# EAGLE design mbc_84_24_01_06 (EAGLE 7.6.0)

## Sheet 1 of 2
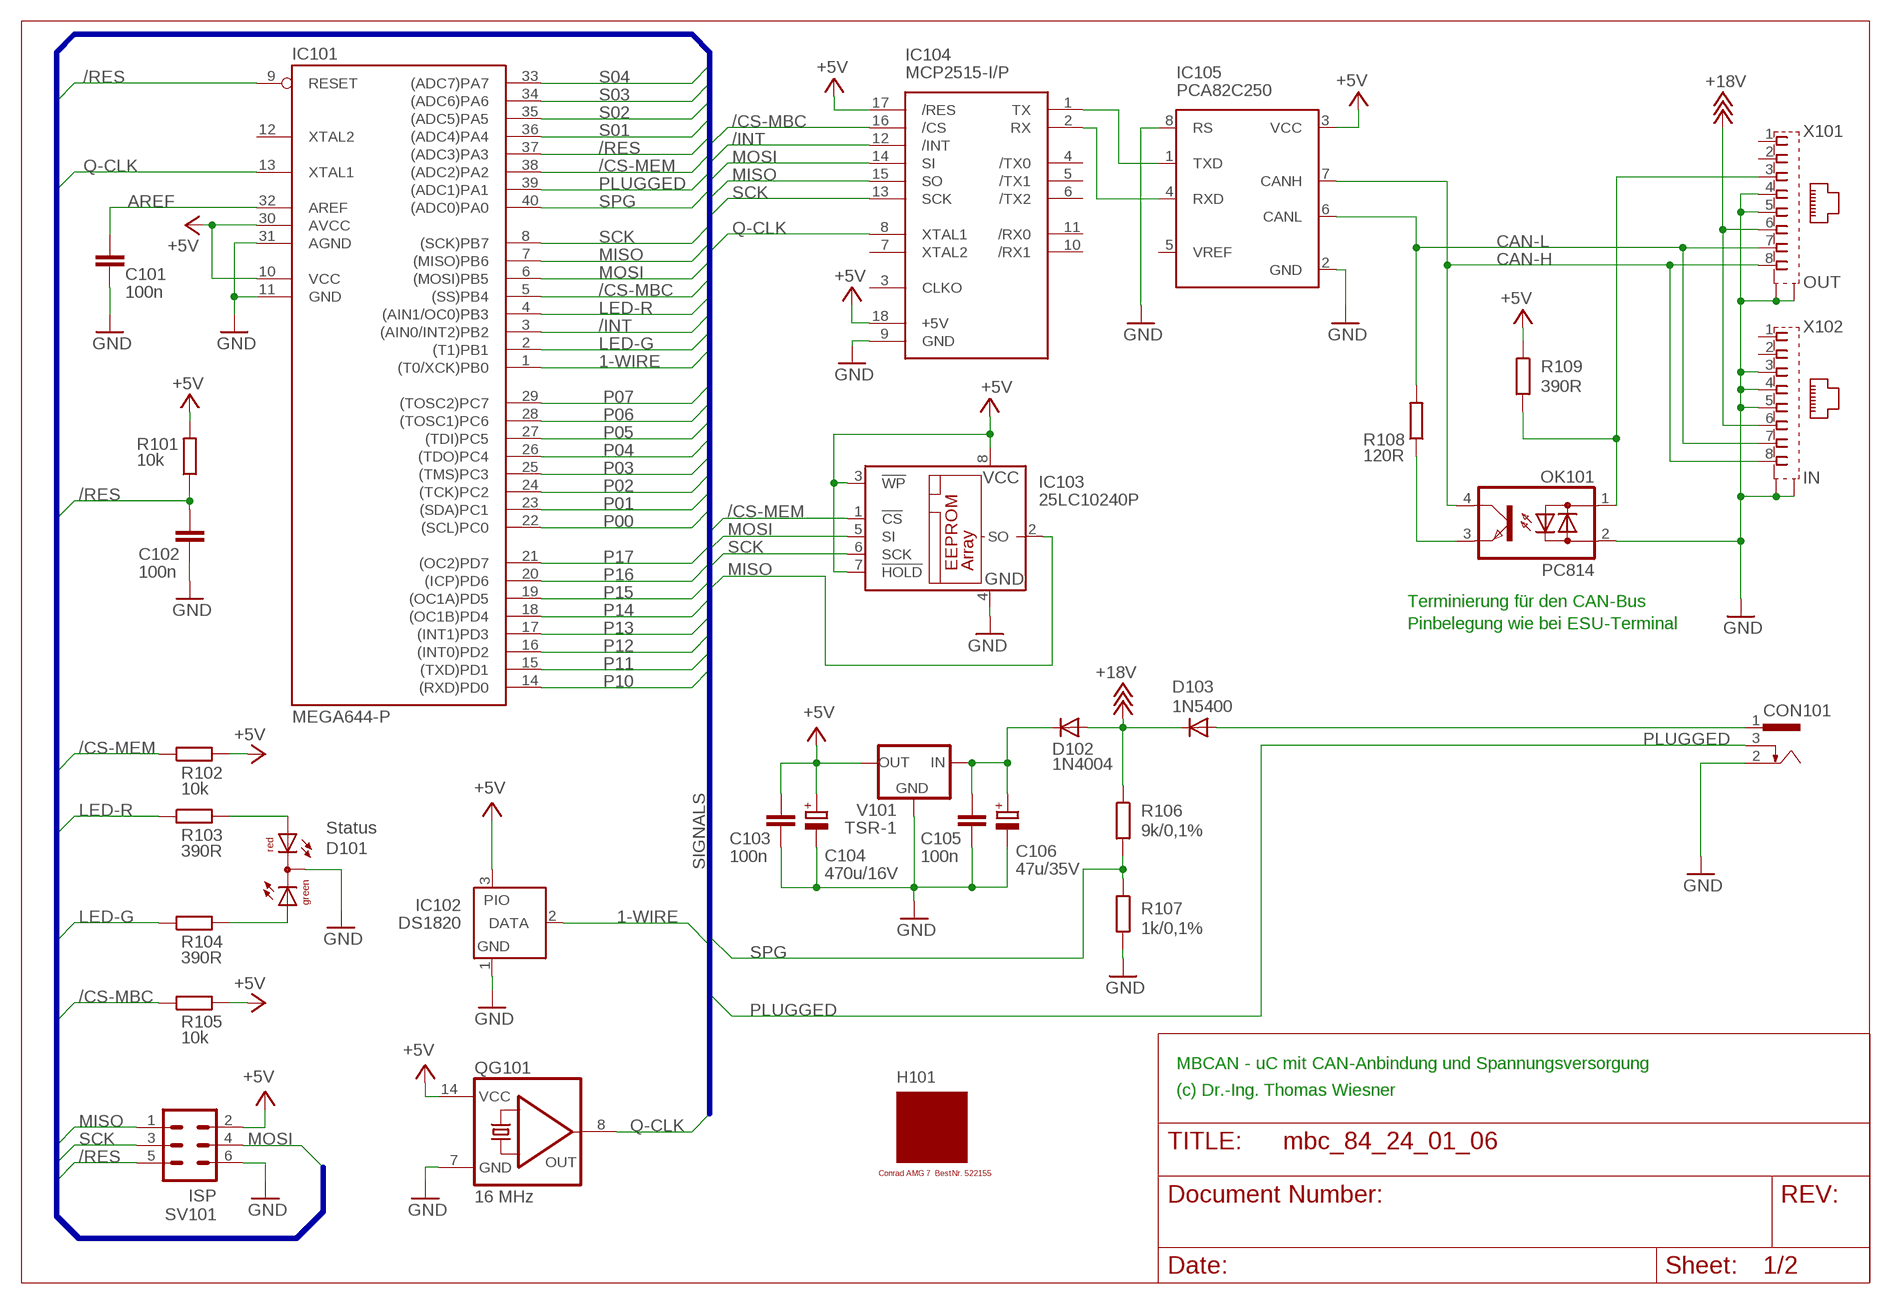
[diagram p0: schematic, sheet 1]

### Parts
C101  100n  C-EU025-025X050  [C025-025X050]
C102  100n  C-EU025-025X050  [C025-025X050]
C103  100n  C-EU025-025X050  [C025-025X050]
C104  470u/16V  CPOL-EUE3.5-8  [E3,5-8]
C105  100n  C-EU025-025X050  [C025-025X050]
C106  47u/35V  CPOL-EUE2.5-7  [E2,5-7]
CON101  POWER-JACK  [POWER-JACK]
D101  Status  DUOLED5MM  [DUOLED5MM]
D102  1N4004  [DO41-10]
D103  1N5400  [DO201-15]
H101  MODULGEHÄUSE-AMG-7  [MODULGEHÄUSE-1]
IC101  MEGA644-P  MEGA323-P  [DIL40]
IC102  DS1820  DS2405  [TO92-]
IC103  25LC10240P  25LC040P  [DIL8]
IC104  MCP2515-I/P  MCP2510-I/P  [DIL18]
IC105  PCA82C250  [DIL08]
OK101  PC814  [DIL04]
QG101  16 MHz  QG5860  [DIL14S]
R101  10k  R-EU_0207/10  [0207/10]
R102  10k  R-EU_0207/10  [0207/10]
R103  390R  R-EU_0207/10  [0207/10]
R104  390R  R-EU_0207/10  [0207/10]
R105  10k  R-EU_0207/10  [0207/10]
R106  9k/0,1%  R-EU_0207/10  [0207/10]
R107  1k/0,1%  R-EU_0207/10  [0207/10]
R108  120R  R-EU_0207/10  [0207/10]
R109  390R  R-EU_0207/10  [0207/10]
SV101  ISP  ML6  [ML6]
V101  TSR-1  [TRACO-TSR-1]
X101  OUT  0446200002  [0446200002]
X102  IN  0446200002  [0446200002]

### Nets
1-WIRE: IC101.1((T0/XCK)PB0) IC102.2(DATA)
+5V: C103.1 C104.+ IC101.10(VCC) IC101.30(AVCC) IC102.3(PIO) IC103.3(!WP) IC103.7(!HOLD) IC103.8(VCC) IC104.17(/RES) IC104.18(+5V) IC105.3(VCC) QG101.14(VCC) R101.2 R102.2 R105.2 R109.1 SV101.2 V101.OUT ; also sheet 2
+18V: D102.A D103.C R106.1 X101.6 X102.6 ; also sheet 2
/CS-MBC: IC101.5((SS)PB4) IC104.16(/CS) R105.1
/CS-MEM: IC101.38((ADC2)PA2) IC103.1(!CS) R102.1
/INT: IC101.3((AIN0/INT2)PB2) IC104.12(/INT)
/RES: C102.1 IC101.9(RESET) IC101.37((ADC3)PA3) R101.1 SV101.5
AREF: C101.1 IC101.32(AREF)
CAN-H: IC105.7(CANH) OK101.4(C) X101.8 X102.8
CAN-L: IC105.6(CANL) R108.2 X101.7 X102.7
GND: C101.2 C102.2 C103.2 C104.- C105.2 C106.- CON101.2 D101.K(C) IC101.11(GND) IC101.31(AGND) IC102.1(GND) IC103.4(GND) IC104.9(GND) IC105.2(GND) IC105.8(RS) OK101.2(AC2) QG101.7(GND) R107.2 SV101.6 V101.GND X101.4 X101.5 X101.S@1(S1) X101.S@2(S2) X102.3 X102.4 X102.5 X102.S@1(S1) X102.S@2(S2) ; also sheet 2
LED-G: IC101.2((T1)PB1) R104.1
LED-R: IC101.4((AIN1/OC0)PB3) R103.1
MISO: IC101.7((MISO)PB6) IC103.2(SO) IC104.15(SO) SV101.1
MOSI: IC101.6((MOSI)PB5) IC103.5(SI) IC104.14(SI) SV101.4
N$1: IC104.1(TX) IC105.1(TXD)
N$2: IC104.2(RX) IC105.4(RXD)
N$3: OK101.3(E) R108.1
N$5: OK101.1(AC1) R109.2 X101.3
N$6: C105.1 C106.+ D102.C V101.IN
N$9: D101.AR R103.2
N$13: D101.AG R104.2
P00: IC101.22((SCL)PC0) ; also sheet 2
P01: IC101.23((SDA)PC1) ; also sheet 2
P02: IC101.24((TCK)PC2) ; also sheet 2
P03: IC101.25((TMS)PC3) ; also sheet 2
P04: IC101.26((TDO)PC4) ; also sheet 2
P05: IC101.27((TDI)PC5) ; also sheet 2
P06: IC101.28((TOSC1)PC6) ; also sheet 2
P07: IC101.29((TOSC2)PC7) ; also sheet 2
P10: IC101.14((RXD)PD0) ; also sheet 2
P11: IC101.15((TXD)PD1) ; also sheet 2
P12: IC101.16((INT0)PD2) ; also sheet 2
P13: IC101.17((INT1)PD3) ; also sheet 2
P14: IC101.18((OC1B)PD4) ; also sheet 2
P15: IC101.19((OC1A)PD5) ; also sheet 2
P16: IC101.20((ICP)PD6) ; also sheet 2
P17: IC101.21((OC2)PD7) ; also sheet 2
PLUGGED: CON101.3 IC101.39((ADC1)PA1)
Q-CLK: IC101.13(XTAL1) IC104.8(XTAL1) QG101.8(OUT)
S01: IC101.36((ADC4)PA4) ; also sheet 2
S02: IC101.35((ADC5)PA5) ; also sheet 2
S03: IC101.34((ADC6)PA6) ; also sheet 2
S04: IC101.33((ADC7)PA7) ; also sheet 2
SCK: IC101.8((SCK)PB7) IC103.6(SCK) IC104.13(SCK) SV101.3
SPG: IC101.40((ADC0)PA0) R106.2 R107.1
V-NETZTEIL1: CON101.1 D103.A
Unconnected: IC101.12(XTAL2) IC104.3(CLKO) IC104.4(/TX0) IC104.5(/TX1) IC104.6(/TX2) IC104.7(XTAL2) IC104.10(/RX1) IC104.11(/RX0) IC105.5(VREF) X101.1 X101.2 X102.1 X102.2

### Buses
SIGNALS

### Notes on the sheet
- Terminierung für den CAN-Bus
- Pinbelegung wie bei ESU-Terminal
- MBCAN - uC mit CAN-Anbindung und Spannungsversorgung
- (c) Dr.-Ing. Thomas Wiesner

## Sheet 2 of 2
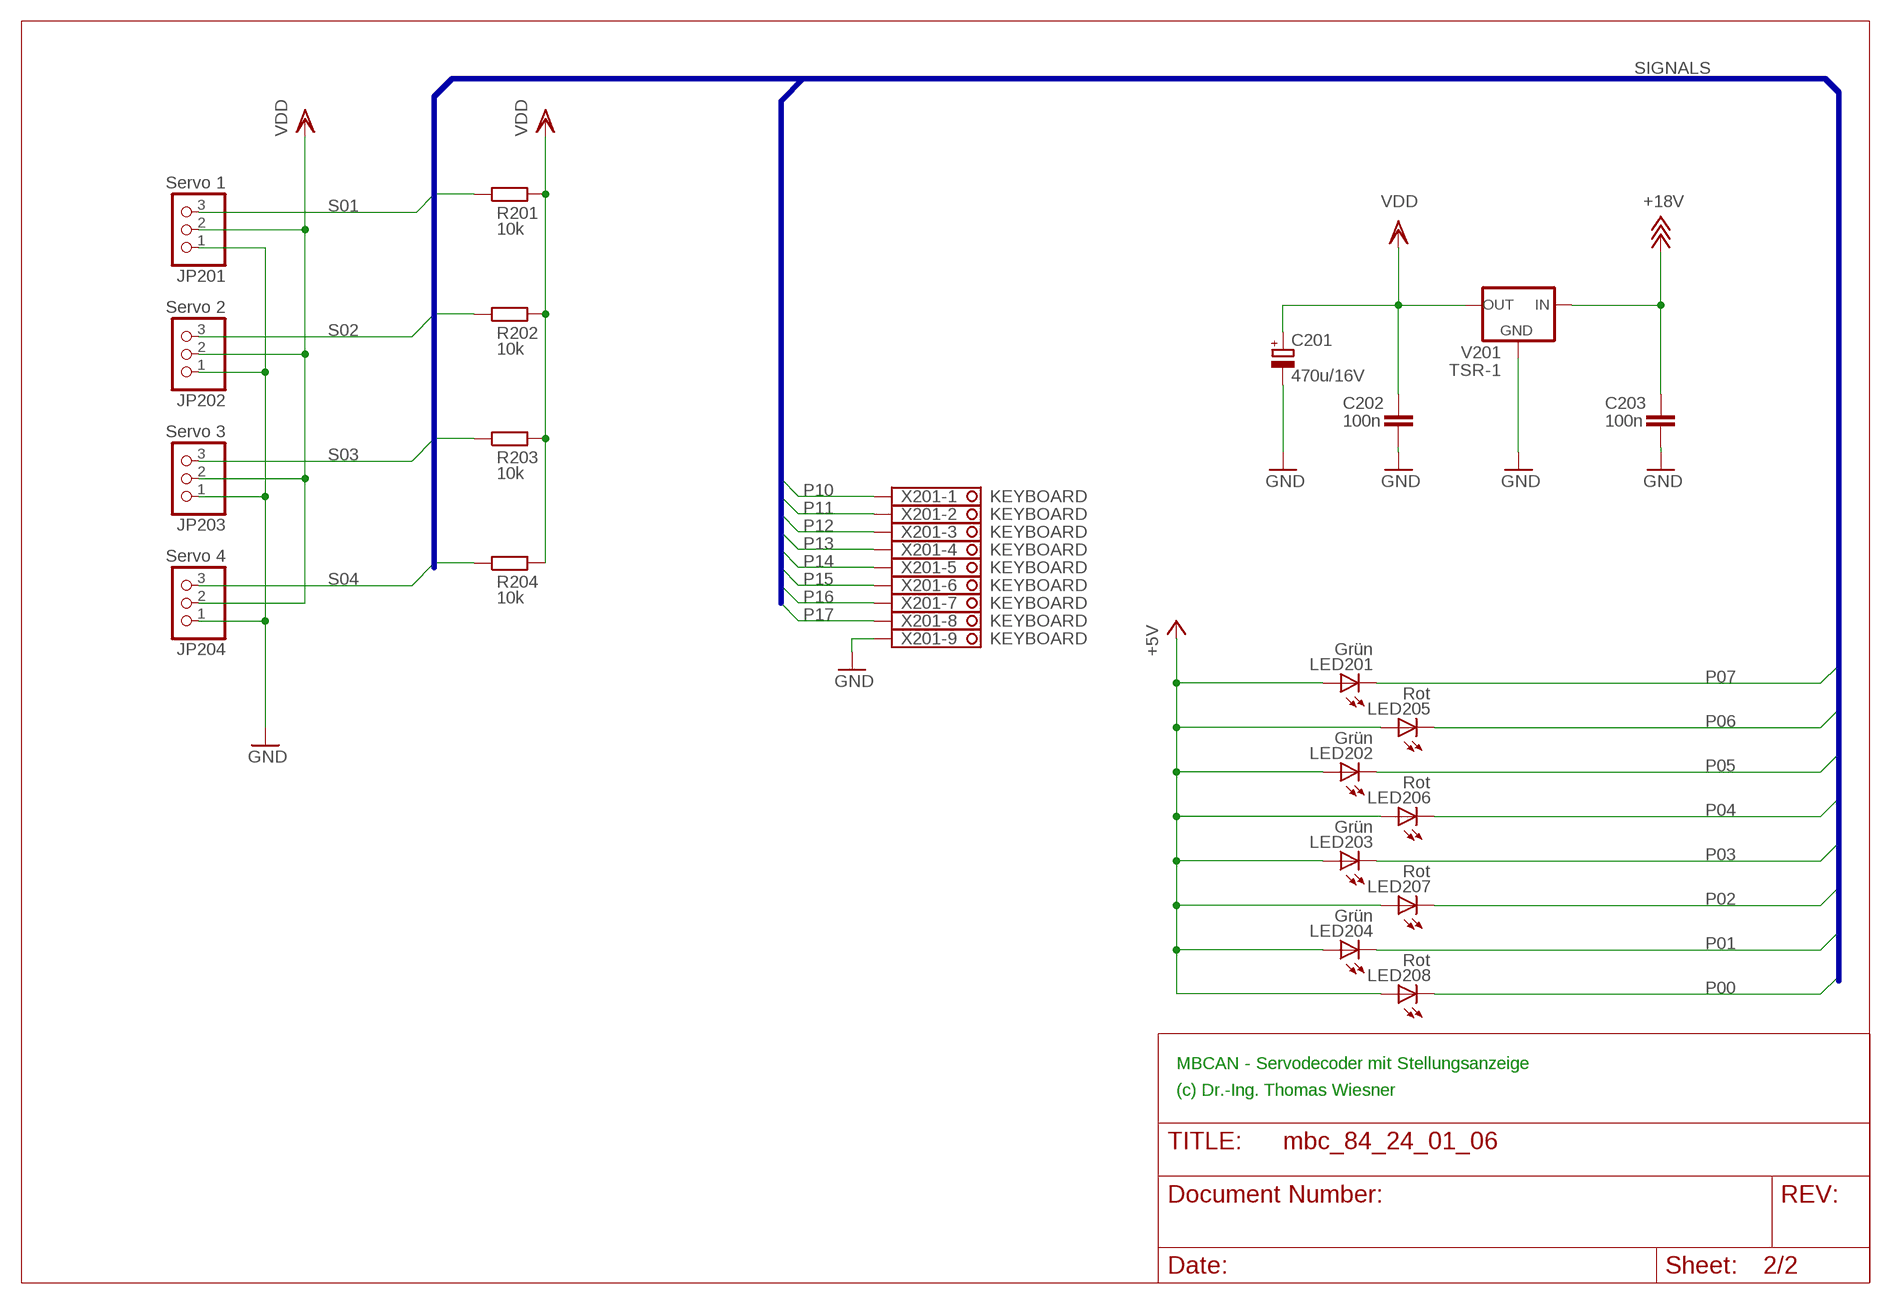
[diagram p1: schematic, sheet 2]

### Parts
C201  470u/16V  CPOL-EUE3.5-8  [E3,5-8]
C202  100n  C-EU025-025X050  [C025-025X050]
C203  100n  C-EU025-025X050  [C025-025X050]
JP201  Servo 1  PINHD-1X3  [1X03]
JP202  Servo 2  PINHD-1X3  [1X03]
JP203  Servo 3  PINHD-1X3  [1X03]
JP204  Servo 4  PINHD-1X3  [1X03]
LED201  Grün  LED3MM  [LED3MM]
LED202  Grün  LED3MM  [LED3MM]
LED203  Grün  LED3MM  [LED3MM]
LED204  Grün  LED3MM  [LED3MM]
LED205  Rot  LED3MM  [LED3MM]
LED206  Rot  LED3MM  [LED3MM]
LED207  Rot  LED3MM  [LED3MM]
LED208  Rot  LED3MM  [LED3MM]
R201  10k  R-EU_0207/10  [0207/10]
R202  10k  R-EU_0207/10  [0207/10]
R203  10k  R-EU_0207/10  [0207/10]
R204  10k  R-EU_0207/10  [0207/10]
V201  TSR-1  [TRACO-TSR-1]
X201  KEYBOARD  1751316  [1751316]

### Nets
+5V: LED201.A LED202.A LED203.A LED204.A LED205.A LED206.A LED207.A LED208.A ; also sheet 1
+18V: C203.1 V201.IN ; also sheet 1
GND: C201.- C202.2 C203.2 JP201.1 JP202.1 JP203.1 JP204.1 V201.GND X201.9 ; also sheet 1
P00: LED208.K(C) ; also sheet 1
P01: LED204.K(C) ; also sheet 1
P02: LED207.K(C) ; also sheet 1
P03: LED203.K(C) ; also sheet 1
P04: LED206.K(C) ; also sheet 1
P05: LED202.K(C) ; also sheet 1
P06: LED205.K(C) ; also sheet 1
P07: LED201.K(C) ; also sheet 1
P10: X201.1 ; also sheet 1
P11: X201.2 ; also sheet 1
P12: X201.3 ; also sheet 1
P13: X201.4 ; also sheet 1
P14: X201.5 ; also sheet 1
P15: X201.6 ; also sheet 1
P16: X201.7 ; also sheet 1
P17: X201.8 ; also sheet 1
S01: JP201.3 R201.1 ; also sheet 1
S02: JP202.3 R202.1 ; also sheet 1
S03: JP203.3 R203.1 ; also sheet 1
S04: JP204.3 R204.1 ; also sheet 1
VDD: C201.+ C202.1 JP201.2 JP202.2 JP203.2 JP204.2 R201.2 R202.2 R203.2 R204.2 V201.OUT

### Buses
SIGNALS

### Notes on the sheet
- MBCAN - Servodecoder mit Stellungsanzeige
- (c) Dr.-Ing. Thomas Wiesner

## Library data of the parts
C101-C103 C105 C202 C203 = rcl:C-EU: CAPACITOR, European symbol
C104 C106 C201 = rcl:CPOL-EU: POLARIZED CAPACITOR, European symbol
CON101 = mbc:POWER-JACK
D101 = led:DUOLED5MM: DUO LED 2 colors, 5 mm, round
D102 = diode:1N4004: DIODE
D103 = diode:1N5400: DIODE
H101 = mbc:MODULGEHÄUSE-AMG-7: Gehäuse
IC101 = atmel:MEGA323-P: MICROCONTROLLER 32 Kbytes FLASH 2 Kbytes SRAM 1 Kbytes EEPROM USART 8-channel 10 bit ADC Source: avr.lbr; OC_FARNELL: unknown; OC_NEWARK: unknown
IC102 = maxim:DS2405: Addressable Switch DALLAS Semiconductor; MF: DALLAS SEMICONDUCTOR; MPN: DS2405; OC_FARNELL: 1188025; OC_NEWARK: 06F4645
IC103 = microchip:25*: Serial EEPROM 4K/ 8K , SPI bus; MF: MICROCHIP; MPN: 25LC040/P; OC_FARNELL: 9758100; OC_NEWARK: 96K4091
IC104 = mbc:MCP2510: BASIC-CAN 2.0a Controller Stand-alone CAN controller von Microchip
IC105 = micro-philips:PCA82C250: CAN CONTROLLER INTERFACE; OC_FARNELL: 3692358; OC_NEWARK: unknown
JP201-JP204 = pinhead:PINHD-1X3: PIN HEADER
LED201-LED208 = led:LED: LED
OK101 = optocoupler:PC814: SHARP OPTO COUPLER; OC_FARNELL: 9707662; OC_NEWARK: unknown
QG101 = crystal:QG5860: CRYSTAL RESONATOR; OC_FARNELL: unknown; OC_NEWARK: unknown
R101-R109 R201-R204 = resistor:R-EU_: RESISTOR, European symbol
SV101 = con-ml:ML6: HARTING; OC_FARNELL: unknown; OC_NEWARK: unknown
V101 V201 = mbc:TSR-1: Spannungsregler Hersteller: TRACO Typ: TSR-1 5V: TSR 1-2450 Spg: 5V Strom: 1A Reichelt TSR 1-2450
X101 X102 = mbc:0446200002: RJ-45 INVERTED MODULAR JACK ASSEMBLY WITH RJ-11 KEEPOUT FEATURE Source: Data sheet MOLEX 0446200002 BUCHSE, RJ45, GESCHIRMT Source: Farnell; MF: MOLEX; MPN: 0446200002; OC_FARNELL: 9251910
X201 = con-phoenix-350:1751316: MKDS 1/ 9-3,5 Printklemme Nennstrom: 10 A Bemessungsspannung: 160 V Raster: 3,5 mm Polzahl: 9 Montageart: Löten Anschlussart: Schraubanschluss Anschlussrichtung vom Leiter zur Platine: 0° Source: http://eshop.phoenixcontact.com .. 1751316.pdf; OC_FARNELL: unknown; OC_NEWARK: unknown

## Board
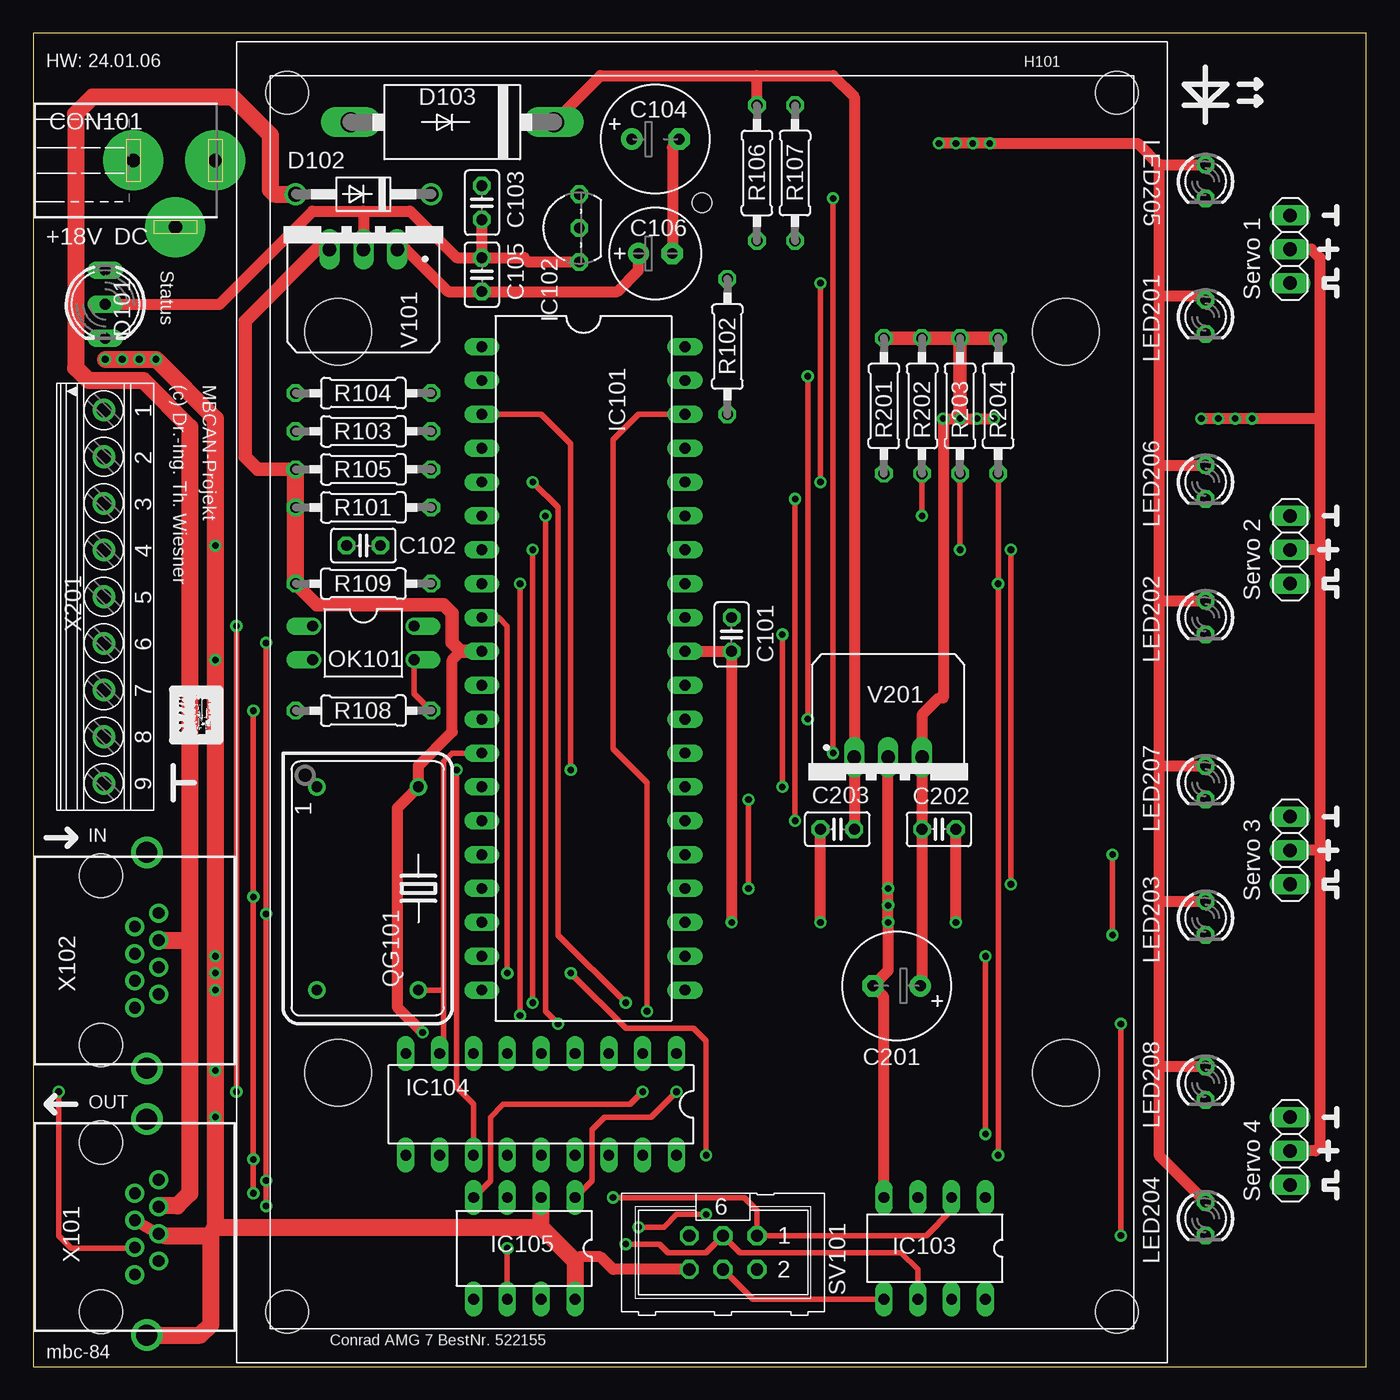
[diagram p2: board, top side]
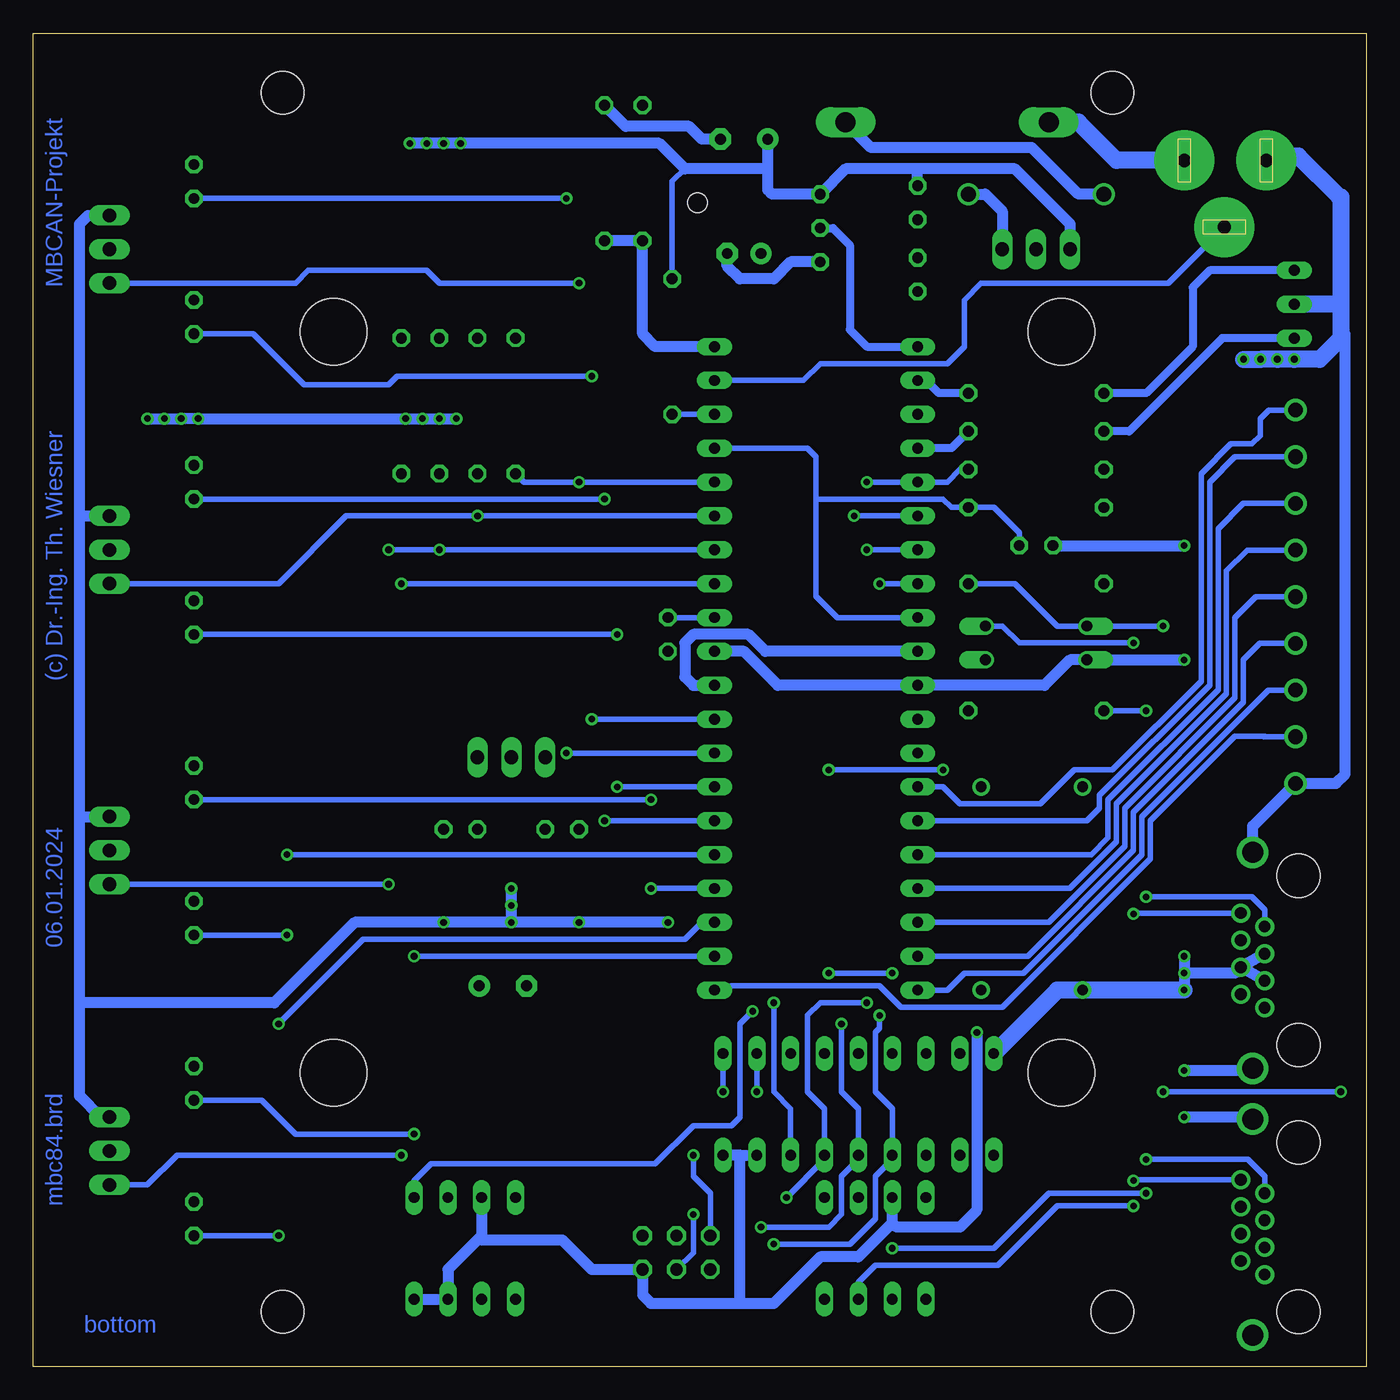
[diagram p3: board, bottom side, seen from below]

Size 100 x 99.99 mm. Coordinates in mm from the lower left corner, seen from the top.
Outline: 0,99.99 0,0 100,0 100,99.99 0,99.99
Copper layers (1*16): Top 0.035mm / dielectric 1.5mm / Bottom 0.035mm
Design rules "default *": minimum track width 10mil, minimum drill 0.5mm, track to track 8mil, track to pad 8mil, pad to pad 8mil, via to via 8mil, smd to smd 8mil, copper to edge 40mil, drill to drill 8mil, minimum pad ring 10mil, minimum via ring 8mil, stop-mask expansion 4mil, vias tented up to drill 0mil, thermal gap 10mil

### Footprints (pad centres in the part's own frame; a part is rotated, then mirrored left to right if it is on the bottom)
C025-025X050 = drill 0.813 octagon: 1 -1.27,0; 2 1.27,0
E3,5-8 = drill 0.813 pad 1.6: + -1.778,0 | drill 0.813 pad 1.6 octagon: - 1.778,0
E2,5-7 = drill 0.813 pad 1.6: + -1.27,0 | drill 0.813 pad 1.6 octagon: - 1.27,0
POWER-JACK = drill 1 pad 4.5: 1 0,6.03; 2 0,-0.12; 3 5,3.03
DUOLED5MM = drill 0.813 long: AG -2.54,0; AR 2.54,0; K 0,0
DO41-10 = drill 1.118: A 5.08,0; C -5.08,0
DO201-15 = drill 1.499 long: A 7.62,0; C -7.62,0
MODULGEHÄUSE-1 = hole 3.2: -45.72,-31.115; -45.72,31.115; 45.72,31.115; 45.72,-31.115 | hole 5: -27.781,-27.305; 27.781,-27.305; -27.781,27.305; 27.781,27.305 | hole 1.5: -37.465,0
DIL40 = drill 0.813 long: 1 -24.13,-7.62; 2 -21.59,-7.62; 3 -19.05,-7.62; 4 -16.51,-7.62; 5 -13.97,-7.62; 6 -11.43,-7.62; 7 -8.89,-7.62; 8 -6.35,-7.62; 9 -3.81,-7.62; 10 -1.27,-7.62; 11 1.27,-7.62; 12 3.81,-7.62; 13 6.35,-7.62; 14 8.89,-7.62; 15 11.43,-7.62; 16 13.97,-7.62; 17 16.51,-7.62; 18 19.05,-7.62; 19 21.59,-7.62; 20 24.13,-7.62; 21 24.13,7.62; 22 21.59,7.62; 23 19.05,7.62; 24 16.51,7.62; 25 13.97,7.62; 26 11.43,7.62; 27 8.89,7.62; 28 6.35,7.62; 29 3.81,7.62; 30 1.27,7.62; 31 -1.27,7.62; 32 -3.81,7.62; 33 -6.35,7.62; 34 -8.89,7.62; 35 -11.43,7.62; 36 -13.97,7.62; 37 -16.51,7.62; 38 -19.05,7.62; 39 -21.59,7.62; 40 -24.13,7.62
TO92- = drill 0.813 octagon: 1 -2.54,0; 2 0,0; 3 2.54,0
DIL8 = drill 0.813 long: 1 -3.81,-3.81; 2 -1.27,-3.81; 3 1.27,-3.81; 4 3.81,-3.81; 5 3.81,3.81; 6 1.27,3.81; 7 -1.27,3.81; 8 -3.81,3.81
DIL18 = drill 0.813 long: 1 -10.16,-3.81; 2 -7.62,-3.81; 3 -5.08,-3.81; 4 -2.54,-3.81 | drill 0.8 long: 5 0,-3.81; 6 2.54,-3.81; 7 5.08,-3.81; 8 7.62,-3.81; 9 10.16,-3.81; 10 10.16,3.81; 11 7.62,3.81; 12 5.08,3.81; 13 2.54,3.81; 14 0,3.81; 15 -2.54,3.81; 16 -5.08,3.81; 17 -7.62,3.81; 18 -10.16,3.81
DIL08 = drill 0.813 long: 1 -3.81,-3.81; 2 -1.27,-3.81; 3 1.27,-3.81; 4 3.81,-3.81; 5 3.81,3.81; 6 1.27,3.81; 7 -1.27,3.81; 8 -3.81,3.81
1X03 = drill 1.016 long: 1 -2.54,0; 2 0,0; 3 2.54,0
LED3MM = drill 0.813 octagon: A -1.27,0; K 1.27,0
DIL04 = drill 0.813 offset: 1 -1.27,-3.81; 2 1.27,-3.81; 3 1.27,3.81; 4 -1.27,3.81
DIL14S = drill 0.813: 1 -7.62,-3.81; 7 7.62,-3.81; 8 7.62,3.81; 14 -7.62,3.81
0207/10 = drill 0.813 octagon: 1 -5.08,0; 2 5.08,0
ML6 = drill 0.914 octagon: 1 -2.54,-1.27; 2 -2.54,1.27; 3 0,-1.27; 4 0,1.27; 5 2.54,-1.27; 6 2.54,1.27
TRACO-TSR-1 = drill 1.016 long: GND 0,2.54; IN -2.54,2.54; OUT 2.54,2.54
0446200002 = drill 0.889 pad 1.422: 1 3.556,2.54; 2 2.54,4.318; 3 1.524,2.54; 4 0.508,4.318; 5 -0.508,2.54; 6 -1.524,4.318; 7 -2.54,2.54; 8 -3.556,4.318 | drill 1.575 pad 2.286: S@1 -8.103,3.429; S@2 8.103,3.429 | hole 3.251: 6.35,0; -6.35,0
1751316 = drill 1.1 pad 1.7: 1 -13.973,-0.1; 2 -10.473,-0.1; 3 -6.973,-0.1; 4 -3.473,-0.1; 5 0.028,-0.1; 6 3.527,-0.1; 7 7.027,-0.1; 8 10.527,-0.1; 9 14.027,-0.1

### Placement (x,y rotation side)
C101  52.39,54.91 270 top
C102  24.77,61.57 180 top
C103  33.66,87.29 270 top
C104  46.67,92.06 0 top
C105  33.66,81.9 90 top
C106  46.67,83.48 0 top
C201  64.77,28.55 180 top
C202  67.94,40.3 0 top
C203  60.33,40.3 180 top
CON101  7.62,90.47 270 top
D101  5.4,79.67 270 top
D102  24.77,87.93 180 top
D103  31.43,93.33 180 top
H101  50.16,49.83 270 top
IC101  41.27,52.37 270 top
IC102  40.96,85.39 90 top
IC103  67.63,8.87 180 top
IC104  38.1,19.66 180 top
IC105  36.83,8.87 180 top
JP201  94.3,83.8 270 top
JP202  94.3,61.26 270 top
JP203  94.3,38.71 270 top
JP204  94.3,16.17 270 top
LED201  87.95,78.72 270 top
LED202  87.95,56.18 270 top
LED203  87.95,33.63 270 top
LED204  87.95,11.09 270 top
LED205  87.95,88.88 270 top
LED206  87.95,66.34 270 top
LED207  87.95,43.79 270 top
LED208  87.95,21.25 270 top
OK101  24.77,54.27 270 top
QG101  25.08,35.86 270 top
R101  24.77,64.43 180 top
R102  52.07,76.5 90 top
R103  24.77,70.15 180 top
R104  24.77,73.01 180 top
R105  24.77,67.29 180 top
R106  54.29,89.52 270 top
R107  57.15,89.52 90 top
R108  24.77,49.19 180 top
R109  24.77,58.72 0 top
R201  63.82,72.05 90 top
R202  66.67,72.05 90 top
R203  69.53,72.05 90 top
R204  72.39,72.05 90 top
SV101  51.75,8.55 180 top
V101  24.77,86.34 180 top
V201  64.14,43.16 0 top
X101  5.08,10.46 270 top
X102  5.08,30.46 270 top
X201  5.4,57.76 270 top

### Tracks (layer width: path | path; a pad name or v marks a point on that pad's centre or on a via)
1-WIRE
  Bottom 0.61: IC102.2 40.01,85.39 38.73,84.12 38.73,77.77 37.47,76.5 IC101.1
+5V  (via drill 0.5)
  Top 0.813: v29.21,25.06 27.3,26.97 27.3,41.89 QG101.14 28.89,45.06 31.43,47.6 31.43,53 32.07,53.64 | LED204.A 84.45,15.86 84.45,22.52 | 84.45,22.52 LED208.A | 84.45,57.45 84.45,45.06 | 84.45,45.06 84.45,34.9 | 84.45,34.9 84.45,22.52 | 84.45,34.9 LED203.A | 84.45,45.06 LED207.A | 84.45,57.45 LED202.A | 84.45,90.15 84.45,80.31 | 84.45,80.31 84.45,67.61 | 84.45,67.61 84.45,57.45 | 84.45,90.15 LED205.A | 84.45,67.61 LED206.A | LED201.A 87.63,80.31 84.45,80.31 | 84.45,90.15 82.87,91.74 v71.75,91.74 v70.48,91.74 v69.22,91.74 v67.94,91.74
  Top 1.016: IC101.10 32.07,53.64 31.43,54.27 31.43,56.49 30.8,57.13 21.27,57.13 R109.1 | V101.OUT 21.27,83.8 15.88,78.4 15.88,68.24 16.83,67.29 R105.2
  Top 1.27: R109.1 R101.2 R105.2
  Bottom 0.406: C104.+ 44.9,89.83 | R102.2 52.07,88.88 51.12,89.83
  Bottom 0.813: 46.99,15.86 IC104.18 | 46.99,15.86 IC104.17 | 46.99,4.74 46.99,15.86 | IC101.10 45.09,53.64 46.35,54.91 50.48,54.91 51.12,54.27 51.12,51.73 50.48,51.1 IC101.30 | 33.66,89.83 26.35,89.83 22.23,85.7 V101.OUT | 33.66,89.83 39.05,89.83 IC102.3 44.58,87.93 44.9,88.25 C104.+ | 44.9,89.83 51.12,89.83 53.02,91.74 v67.94,91.74 v69.22,91.74 v70.48,91.74 v71.75,91.74 | 35.56,10.78 38.1,8.24 40.96,8.24 44.45,4.74 46.99,4.74 | 35.56,10.78 IC105.3 | v29.21,25.06 29.21,11.73 30.48,10.46 35.24,10.46 35.56,10.78 | 46.99,4.74 53.66,4.74 54.29,5.38 SV101.2 58.1,7.28 60.33,9.51 66.36,9.51 IC103.3 66.36,9.82 68.9,7.28 IC103.7 IC103.8 | C103.1 33.66,89.83
+18V
  Top 0.813: D103.C 42.55,96.82 54.29,96.82 | 54.29,96.82 60.01,96.82 61.59,95.23 V201.IN C203.1 | R106.1 54.29,96.82
  Top 1.27: 11.75,32.05 11.75,70.47 8.26,73.96 4.13,73.96 3.17,74.91 3.17,93.96 4.45,95.23 14.92,95.23 17.78,92.37 17.78,88.25 18.1,87.93 D102.A | 11.75,32.05 11.75,13 10.79,12.04 9.46,12.04 X101.6 | X102.6 11.68,31.98 11.75,32.05
  Bottom 0.813: D102.A 21.59,87.93 25.08,91.42 37.15,91.42 D103.C
/CS-MBC  (via drill 0.5)
  Top 0.406: v37.47,66.34 39.37,64.43 39.37,32.36 v44.45,27.29
  Bottom 0.406: v37.47,66.34 IC101.5 31.43,66.34 30.48,67.29 R105.1 | v44.45,27.29 44.45,20.62 43.18,19.35 IC104.16
/CS-MEM  (via drill 0.5)
  Top 0.406: v46.04,26.65 46.04,43.79 43.5,46.33 43.5,69.51 45.4,71.42 IC101.38
  Bottom 0.406: R102.1 IC101.38 | IC103.1 71.44,13.95 70.17,15.22 53.34,15.22 50.48,18.08 47.62,18.08 46.99,18.71 46.99,25.7 v46.04,26.65
/INT  (via drill 0.5)
  Top 0.406: IC104.12 33.02,19.66 31.75,20.93 v31.75,44.75 | v40.32,44.75 40.32,69.2 38.1,71.42 IC101.3
  Bottom 0.406: v31.75,44.75 v40.32,44.75
/RES  (via drill 0.5)
  Top 0.406: v35.56,29.51 35.56,55.54 34.92,56.18 IC101.9 | v40.32,29.51 44.45,25.38 49.53,25.38 50.48,24.43 v50.48,15.86
  Bottom 0.406: IC101.37 41.91,68.88 41.27,68.24 41.27,65.07 | 41.27,65.07 41.27,57.76 39.69,56.18 IC101.9 | v35.56,29.51 v40.32,29.51 | v50.48,15.86 50.48,14.27 49.21,13 SV101.5 | 41.27,65.07 31.75,65.07 31.11,64.43 R101.1 27.94,64.43 26.04,62.53 C102.1
AREF
  Bottom 0.406: IC101.32 C101.1
CAN-H  (via drill 0.5)
  Top 0.406: v17.46,54.27 v17.46,33.95 v17.46,13.95 v17.46,12.04
  Bottom 0.406: X101.8 17.4,14.01 v17.46,13.95 | v17.46,54.27 26.04,54.27 27.3,55.54 OK101.4 | v17.46,12.04 23.18,12.04 27.62,7.6 36.83,7.6 38.1,6.33 IC105.7 | X102.8 17.4,34.02 v17.46,33.95
CAN-L  (via drill 0.5)
  Top 0.406: v16.51,49.19 v16.51,35.22 v16.51,15.54 v16.51,13 | v35.56,8.87 IC105.6
  Bottom 0.406: R108.2 v16.51,49.19 | v16.51,13 23.81,13 27.94,8.87 v35.56,8.87 | X101.7 7.62,14.27 8.89,15.54 v16.51,15.54 | X102.7 7.62,34.27 8.57,35.22 v16.51,35.22
GND  (via drill 0.5)
  Top 0.406: C104.- 48.45,91.93
  Top 0.813: 24.77,86.66 V101.GND | 24.77,86.66 28.26,86.66 31.75,83.17 C105.2 | C105.2 36.83,83.17 37.15,82.85 IC102.1 | D101.K 13.97,79.67 20.95,86.66 24.77,86.66 | 48.45,91.93 47.94,91.42 C106.- | IC101.31 C101.2 v52.39,33.32 | v59.05,33.32 C203.2 | v69.22,33.32 C202.2 | V201.GND v64.14,35.86 v64.14,34.59 v64.14,33.32 64.14,29.7 C201.- 63.82,27.73 IC103.4 | SV101.6 43.5,7.28 42.55,8.24 40.96,8.24 40.64,7.92 | X101.5 X101.4 | C105.2 C103.2
  Top 1.27: 13.65,10.46 v13.65,18.71 v13.65,22.21 v13.65,28.24 v13.65,29.51 v13.65,30.78 v13.65,53 v13.65,61.57 13.65,71.1 v9.21,75.55 v5.4,75.55 | 13.65,10.46 13.18,9.66 13.34,9.82 | IC105.8 40.64,7.92 38.1,10.46 | 38.1,10.46 IC105.2 | 13.65,10.46 38.1,10.46 | X101.S@2 12.54,2.35 13.34,3.15 13.34,9.82 | X101.4 9.84,9.82 13.34,9.82
  Bottom 0.61: 1.59,77.45 1.91,77.77
  Bottom 0.813: IC101.31 46.67,53.64 44.13,51.1 IC101.11 24.13,51.1 22.23,53 OK101.2 v13.65,53 | v52.39,33.32 v59.05,33.32 v64.14,33.32 | 96.52,27.29 81.92,27.29 75.88,33.32 v69.22,33.32 v64.14,33.32 | JP204.1 94.93,18.71 96.52,20.3 96.52,27.29 | 96.52,27.29 96.52,41.25 | 96.52,41.25 JP203.1 | 96.52,41.25 96.52,63.8 | 96.52,63.8 JP202.1 | 96.52,63.8 96.52,85.7 95.89,86.34 JP201.1 | v64.14,33.32 v64.14,34.59 v64.14,35.86 | 1.59,77.45 1.59,44.43 2.28,43.74 X201.9 8.51,40.53 X102.S@1 | C102.2 v13.65,61.57 | X101.S@1 8.66,18.71 v13.65,18.71 | X102.S@2 8.66,22.21 v13.65,22.21 | X102.5 X102.4 | X102.3 X102.4 | X102.4 9.84,29.51 v13.65,29.51 | v13.65,30.78 v13.65,28.24 | C104.- 49.85,92.06 50.8,93.01 55.56,93.01 R107.2 | IC102.1 43.18,82.85 44.45,81.58 46.99,81.58 47.94,82.53 C106.-
  Bottom 1.27: 1.91,79.67 1.91,87.73 2.02,87.73 5.08,90.79 7.18,90.79 CON101.2 | 1.91,79.67 D101.K | 1.91,79.67 1.91,77.77 1.91,77.13 3.49,75.55 v5.4,75.55 v6.67,75.55 v7.94,75.55 v9.21,75.55 | v13.65,28.24 QG101.7 23.18,28.24 IC104.9
LED-G
  Bottom 0.61: R104.1 32.07,73.01 33.02,73.96 IC101.2
LED-R
  Bottom 0.61: IC101.4 31.11,68.88 R103.1
MISO  (via drill 0.5)
  Top 0.406: v37.47,61.26 v37.47,27.29 | IC103.2 68.9,11.73 66.99,9.82 SV101.1 54.29,11.73 53.34,12.68 v43.5,12.68
  Bottom 0.406: IC101.7 v37.47,61.26 | v37.47,27.29 40.96,27.29 41.91,26.33 41.91,20.62 40.64,19.35 IC104.15 40.64,15.54 v43.5,12.68
MOSI  (via drill 0.5)
  Top 0.406: v38.42,63.8 38.42,26.65 v39.37,25.7 | IC103.5 53.98,5.06 SV101.4 | v45.4,10.46 47.31,10.46 48.26,11.41 v50.48,11.41
  Bottom 0.406: IC101.6 v38.42,63.8 | v39.37,25.7 39.37,20.62 38.1,19.35 IC104.14 38.1,15.54 39.37,14.27 39.37,11.41 40.32,10.46 v45.4,10.46 | v50.48,11.41 50.48,8.55 SV101.4
N$1  (via drill 0.5)
  Top 0.406: v48.26,20.62 46.35,18.71 42.86,18.71 41.91,17.76 41.91,13.95 IC105.1
  Bottom 0.406: v48.26,20.62 IC104.1
N$2  (via drill 0.5)
  Top 0.406: v45.72,20.62 44.77,19.66 35.24,19.66 34.29,18.71 34.29,13.95 IC105.4
  Bottom 0.406: v45.72,20.62 IC104.2
N$3
  Top 0.406: OK101.3 28.57,50.46 R108.1
N$5  (via drill 0.5)
  Top 0.406: v15.24,55.54 v15.24,20.62 | v1.91,20.62 1.91,9.82 2.86,8.87 7.56,8.87 X101.3
  Bottom 0.406: R109.2 26.35,58.72 23.18,55.54 OK101.1 v15.24,55.54 | v15.24,20.62 v1.91,20.62
N$6
  Top 0.813: V101.IN 27.94,83.8 31.11,80.62 C105.1 43.81,80.62 45.4,82.21 C106.+
  Bottom 0.813: V101.IN 27.3,86.66 28.57,87.93 D102.C
N$9
  Bottom 0.61: R103.2 17.78,70.15 10.79,77.13 D101.AR
N$13
  Bottom 0.61: R104.2 16.51,73.01 13.02,76.5 13.02,80.94 11.75,82.21 D101.AG
P00  (via drill 0.5)
  Top 0.406: v71.44,17.44 v71.44,30.78
  Bottom 0.406: LED208.K 82.87,19.98 80.33,17.44 v71.44,17.44 | v71.44,30.78 IC101.22
P01  (via drill 0.5)
  Top 0.406: v81.6,25.7 v81.6,9.82
  Bottom 0.406: IC101.23 49.85,33.32 51.12,32.05 75.25,32.05 v81.6,25.7 | v81.6,9.82 LED204.K
P02  (via drill 0.5)
  Top 0.406: v53.66,42.52 v53.66,35.86
  Bottom 0.406: LED207.K v53.66,42.52 | v53.66,35.86 IC101.24
P03  (via drill 0.5)
  Top 0.406: v80.96,38.4 v80.96,32.36
  Bottom 0.406: IC101.25 v80.96,38.4 | v80.96,32.36 LED203.K
P04  (via drill 0.5)
  Top 0.406: v57.15,65.07 v57.15,40.94
  Bottom 0.406: LED206.K v57.15,65.07 | v57.15,40.94 IC101.26
P05  (via drill 0.5)
  Top 0.406: v56.2,54.91 v56.2,43.48
  Bottom 0.406: LED202.K v56.2,54.91 | v56.2,43.48 IC101.27
P06  (via drill 0.5)
  Top 0.406: v60.01,87.61 v60.01,46.02
  Bottom 0.406: LED205.K v60.01,87.61 | v60.01,46.02 IC101.28
P07  (via drill 0.5)
  Top 0.406: v58.1,74.28 v58.1,48.56
  Bottom 0.406: LED201.K 83.5,77.45 79.69,73.64 73.34,73.64 72.71,74.28 v58.1,74.28 | v58.1,48.56 IC101.29
P10
  Bottom 0.406: X201.1 7.3,71.74 7.94,71.1 7.94,69.83 8.57,69.2 10.16,69.2 12.38,66.97 12.38,51.41 19.05,44.75 21.91,44.75 24.45,42.21 30.48,42.21 31.75,43.48 IC101.14
P11
  Bottom 0.406: X201.2 9.85,68.24 11.75,66.34 11.75,51.1 20,42.84 20,41.89 20.95,40.94 IC101.15
P12
  Bottom 0.406: X201.3 9.22,64.74 11.11,62.84 11.11,50.78 19.37,42.52 19.37,39.67 20.64,38.4 IC101.16
P13
  Bottom 0.406: X201.4 8.91,61.24 10.48,59.67 10.48,50.46 18.73,42.21 18.73,39.35 22.23,35.86 IC101.17
P14
  Bottom 0.406: X201.5 8.28,57.74 9.84,56.18 9.84,50.14 18.1,41.89 18.1,39.03 23.81,33.32 IC101.18
P15
  Bottom 0.406: X201.6 7.97,54.24 9.21,53 9.21,49.83 17.46,41.57 17.46,38.71 25.4,30.78 IC101.19
P16
  Bottom 0.406: X201.7 7.34,50.74 16.83,41.25 16.83,38.4 25.72,29.51 30.16,29.51 31.43,28.24 IC101.20
P17
  Bottom 0.406: X201.8 7.67,47.24 7.62,47.29 9.84,47.29 16.19,40.94 16.19,38.08 27.3,26.97 34.92,26.97 36.51,28.55 47.62,28.55 47.94,28.24 IC101.21
PLUGGED
  Bottom 0.406: IC101.39 42.23,73.96 40.96,75.23 31.43,75.23 30.16,76.5 30.16,79.99 28.89,81.26 14.86,81.26 CON101.3
Q-CLK
  Top 0.406: IC101.13 31.43,46.02 30.8,45.38 30.8,28.24 | 30.8,28.24 30.8,23.79 IC104.8 | 30.8,28.24 QG101.8
S01  (via drill 0.5)
  Top 0.406: v59.05,81.26 v59.05,66.34
  Bottom 0.406: JP201.3 80.33,81.26 79.38,82.21 70.48,82.21 69.53,81.26 v59.05,81.26 | IC101.36 v59.05,66.34 63.18,66.34 R201.1
S02  (via drill 0.5)
  Top 0.406: R202.1 v66.67,63.8
  Bottom 0.406: JP202.3 81.6,58.72 76.52,63.8 v66.67,63.8 IC101.35
S03  (via drill 0.5)
  Top 0.406: v73.34,36.17 v73.34,61.26 | R203.1 v69.53,61.26
  Bottom 0.406: JP203.3 v73.34,36.17 | v73.34,61.26 v69.53,61.26 IC101.34
S04  (via drill 0.5)
  Top 0.406: v72.39,15.86 v72.39,58.72 R204.1
  Bottom 0.406: IC101.33 v72.39,58.72 | v72.39,15.86 89.22,15.86 91.44,13.63 JP204.3
SCK  (via drill 0.5)
  Top 0.406: v36.51,58.72 v36.51,26.33 | IC103.6 66.36,7.28 65.09,8.55 53.02,8.55 SV101.3 50.48,8.55 47.62,8.55 46.99,9.19 v44.45,9.19
  Bottom 0.406: IC101.8 v36.51,58.72 | v36.51,26.33 36.51,25.38 36.83,25.06 36.83,20.62 35.56,19.35 IC104.13 35.56,15.54 36.83,14.27 36.83,11.09 38.73,9.19 v44.45,9.19
SPG
  Bottom 0.813: IC101.40 53.34,76.5 54.29,77.45 R106.2 R107.1
V-NETZTEIL1
  Bottom 1.27: CON101.1 18.73,90.47 21.59,93.33 D103.A
VDD  (via drill 0.5)
  Top 0.813: JP204.2 96.2,16.17 96.52,16.49 96.52,38.71 | 96.52,71.1 96.52,83.17 95.89,83.8 JP201.2 | 96.52,71.1 96.52,61.26 | 96.52,61.26 JP202.2 | 96.52,38.71 JP203.2 | 96.52,61.26 96.52,38.71 | 96.52,71.1 v91.44,71.1 v87.63,71.1 | v72.07,71.1 v70.8,71.1 v69.53,71.1 v68.26,71.1 68.26,50.14 67.94,50.14 66.67,48.88 V201.OUT C202.1 66.67,28.55 C201.+
  Top 1.016: R201.2 R202.2 R203.2 | R204.2 R203.2 | R203.2 v69.53,71.1
  Bottom 0.813: v68.26,71.1 v69.53,71.1 v70.8,71.1 v72.07,71.1 v87.63,71.1 v88.9,71.1 v90.17,71.1 v91.44,71.1

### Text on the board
Bottom: MBCAN-Projekt | (c) Dr.-Ing. Th. Wiesner | 06.01.2024 | mbc84.brd | bottom
tNames: HW: 24.01.06 | +18V | DC | Status | (c) Dr.-Ing. Th. Wiesner | MBCAN-Projekt | IN | OUT | mbc-84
